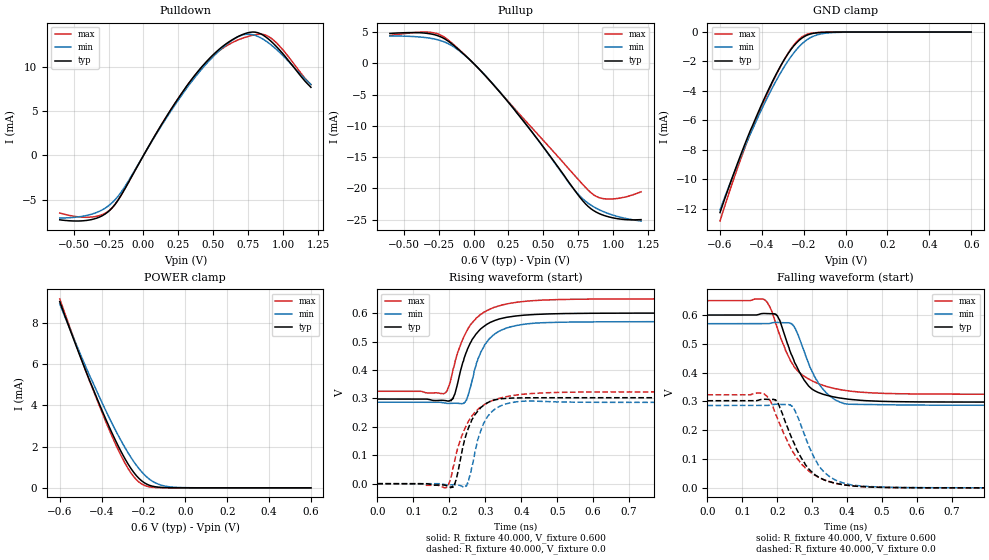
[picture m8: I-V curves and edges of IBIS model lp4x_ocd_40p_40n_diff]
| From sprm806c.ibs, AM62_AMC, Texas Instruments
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|   Model lp4x_ocd_40p_40n_diff
[Model] lp4x_ocd_40p_40n_diff
Model_type I/O
Polarity   Non-Inverting
Enable   Active-High
Vinl =  0.0V
Vinh =  0.900V
Vmeas =  0.600V
C_comp   1.772pF   1.574pF   2.047pF
[Model Spec]
Vinh   0.900V   0.900V   0.900V
Vinl   0.0V   0.0V   0.0V
Vmeas   0.600V   NA   NA
[Temperature Range]   25.000   0.125k   -40.000
[Voltage Range]   0.600V   0.570V   0.650V
[Pullup Reference]   0.600V   0.570V   0.650V
[Pulldown Reference]   0.0V   0.0V   0.0V
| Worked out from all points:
|   slope of the pulldown table from 0 to 0.09 V, typ, clamps not added: 36.7 ohm
|   slope of the pullup table from 0 to 0.09 V, typ, clamps not added: 42.8 ohm
|   GND clamp passes 1 mA (typ) near -0.25 V on its own axis
|   POWER clamp passes 1 mA (typ) near -0.26 V on its own axis
|   rising waveform, R_fixture 40.000, V_fixture 0.600: 20-80 % time 59.5ps typ, 54.7ps min, 68.8ps max; typ from 0.298 V to 0.6 V
|   rising waveform, R_fixture 40.000, V_fixture 0.0: 20-80 % time 43.8ps typ, 40.4ps min, 64.1ps max; typ from 0 V to 0.302 V
|   falling waveform, R_fixture 40.000, V_fixture 0.600: 20-80 % time 68.4ps typ, 65.2ps min, 81.6ps max; typ from 0.6 V to 0.298 V
|   falling waveform, R_fixture 40.000, V_fixture 0.0: 20-80 % time 74.9ps typ, 68.1ps min, 90.2ps max; typ from 0.302 V to 0 V
[Pulldown]
|Voltage   I(typ)   I(min)   I(max)
-600mV    -7.251mA   -7.047mA   -6.479mA
-392mV    -7.283mA   -6.702mA   -6.959mA
-240mV    -6.158mA   -5.537mA   -6.133mA
-145mV    -4.078mA   -3.792mA   -4.063mA
120mV     3.243mA    3.131mA    3.229mA
328mV     8.216mA    7.975mA    8.184mA
499mV     11.35mA    11.14mA    11.23mA
669mV     13.34mA    13.31mA    12.96mA
802mV     13.89mA    13.52mA    13.61mA
897mV     13.1mA     12.68mA    13.4mA
992mV     11.59mA    11.37mA    12.03mA
1.2V      7.68mA     7.991mA    7.987mA
[Pullup]
|Voltage   I(typ)   I(min)   I(max)
-600mV    4.81mA     4.404mA    4.474mA
-278mV    4.589mA    3.904mA    4.871mA
-202mV    3.866mA    3.377mA    4.097mA
-107mV    2.214mA    2.104mA    2.298mA
44.21mV   -1.008mA   -999.9uA   -1.029mA
234mV     -5.817mA   -5.774mA   -5.74mA
461mV     -12.23mA   -12.25mA   -11.38mA
707mV     -19.78mA   -19.83mA   -17.51mA
840mV     -23.26mA   -22.68mA   -20.69mA
897mV     -24.02mA   -23.4mA    -21.47mA
973mV     -24.6mA    -24.1mA    -21.72mA
1.2V      -25.02mA   -25.24mA   -20.56mA
[GND_clamp]
|Voltage   I(typ)   I(min)   I(max)
-600mV    -12.26mA   -12.07mA   -12.83mA
-535mV    -9.631mA   -9.657mA   -9.999mA
-483mV    -7.674mA   -7.84mA    -7.926mA
-457mV    -6.749mA   -6.974mA   -6.957mA
-378mV    -4.198mA   -4.571mA   -4.306mA
-326mV    -2.706mA   -3.156mA   -2.747mA
-287mV    -1.735mA   -2.22mA    -1.722mA
-248mV    -949.8uA   -1.424mA   -887.7uA
-209mV    -414uA     -806.5uA   -336.6uA
-157mV    -95.46uA   -302uA     -61.62uA
-78.26mV  -9.128uA   -53.02uA   -8.175uA
600mV     0A         0A         0A
[POWER_clamp]
|Voltage   I(typ)   I(min)   I(max)
-600mV    9.037mA    8.928mA    9.175mA
-457mV    5.197mA    5.441mA    5.166mA
-352mV    2.698mA    3.164mA    2.544mA
-313mV    1.878mA    2.4mA      1.683mA
-274mV    1.164mA    1.707mA    946.8uA
-248mV    770.4uA    1.297mA    560.4uA
-222mV    461.7uA    938.4uA    283.8uA
-196mV    245.9uA    638.9uA    120.5uA
-157mV    79.31uA    316.3uA    23.58uA
-117mV    22.67uA    136.3uA    6.088uA
-78.26mV  6.714uA    54.46uA    1.894uA
600mV     0A         0A         0A
[Ramp]
| variable   typ   min   max
dV/dt_r   0.181/43.760p   0.172/39.810p   0.194/64.335p
dV/dt_f   0.182/68.438p   0.170/65.045p   0.195/81.489p
R_load = 40.000
[Rising Waveform]
R_fixture= 40.000
V_fixture= 0.600
V_fixture_min= 0.570
V_fixture_max= 0.650
|time   V(typ)   V(min)   V(max)
0s        297.7mV    286.6mV    325.1mV
187ps     292.7mV    283.5mV    317.8mV
195ps     290.9mV    282.2mV    329.2mV
210ps     298.5mV    282.9mV    399.1mV
241ps     440.3mV    283.2mV    518.2mV
252ps     477.3mV    308.4mV    545.7mV
280ps     534.9mV    439.9mV    587.5mV
310ps     564.4mV    507.9mV    612mV
426ps     594.2mV    563.3mV    643.1mV
3ns       600mV      569.9mV    650mV
[Rising Waveform]
R_fixture= 40.000
V_fixture= 0.0
V_fixture_min= 0.0
V_fixture_max= 0.0
|time   V(typ)   V(min)   V(max)
0s        38.54uV    204.1uV    38.35uV
193ps     -7.485mV   -3.865mV   -12.63mV
215ps     -2.737mV   -3.064mV   80.39mV
244ps     161.4mV    -12.07mV   195.6mV
258ps     210.2mV    28.82mV    230mV
271ps     242.3mV    109.9mV    251.6mV
306ps     284.6mV    235.8mV    284.3mV
353ps     299.7mV    278.8mV    304.7mV
419ps     302.1mV    290.8mV    316.2mV
3ns       302.5mV    286.1mV    323.1mV
[Falling Waveform]
R_fixture= 40.000
V_fixture= 0.600
V_fixture_min= 0.570
V_fixture_max= 0.650
|time   V(typ)   V(min)   V(max)
0s        600mV      569.9mV    650mV
164ps     605.4mV    569.9mV    653.3mV
200ps     598.2mV    574.4mV    556.5mV
239ps     467.2mV    571.4mV    439.1mV
256ps     421mV      542.3mV    409.2mV
286ps     359.6mV    444.1mV    380.7mV
331ps     325.1mV    342.6mV    356mV
376ps     312.5mV    299.7mV    342.1mV
429ps     304.9mV    289.9mV    333.3mV
3ns       297.7mV    286.6mV    325.1mV
[Falling Waveform]
R_fixture= 40.000
V_fixture= 0.0
V_fixture_min= 0.0
V_fixture_max= 0.0
|time   V(typ)   V(min)   V(max)
0s        302.5mV    286.1mV    323mV
162ps     307.8mV    286.1mV    326.7mV
179ps     306.9mV    287.1mV    304.8mV
199ps     300.4mV    290.5mV    246.2mV
237ps     187.2mV    289mV      142.4mV
251ps     147.7mV    267.6mV    112.8mV
280ps     81.48mV    180.1mV    70.27mV
325ps     33.37mV    67.31mV    32.68mV
416ps     6.717mV    9.856mV    6.912mV
3ns       38.01uV    202.3uV    37.78uV
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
